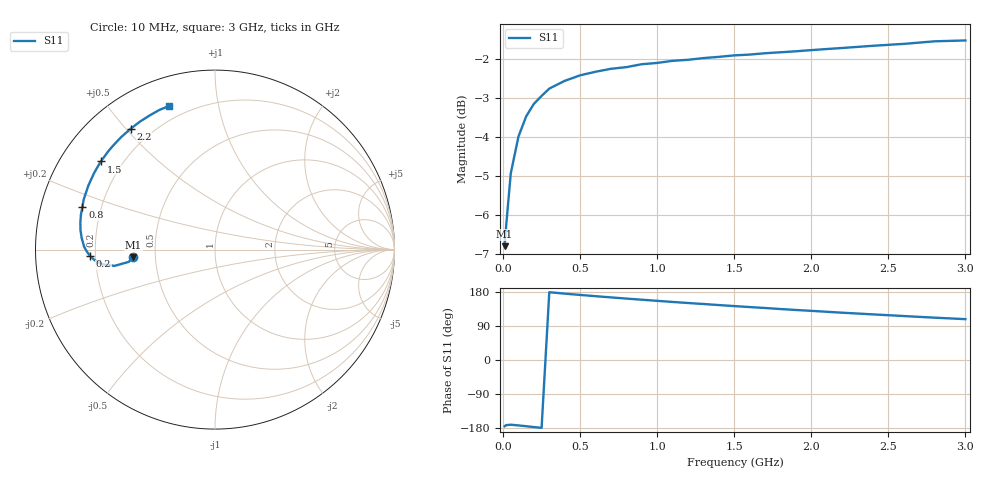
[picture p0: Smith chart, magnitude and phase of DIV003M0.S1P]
! SIEMENS Small Signal Semiconductors
! BAV99
! Silicon Switching Diode in SOT23
! IF = 3 mA
! S-Parameters:  May  1995
# GHz  S  MA  R  50
!  f  S11
! GHz  MAG  ANG
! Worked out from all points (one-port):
!   30 points, 10 MHz to 3 GHz, reference 50 ohm
!   lowest |S11| = -6.8 dB at 10 MHz (marker M1), VSWR 2.69, Z = 18.6 - j1.96 ohm
!   |S11| at or under -10 dB: nowhere
!   S11 on the Smith chart (normalised r, x): 10 MHz: 0.37, -0.04; 200 MHz: 0.18, -0.03; 800 MHz: 0.13, +0.15; 1.5 GHz: 0.12, +0.34; 2.2 GHz: 0.12, +0.52; 3 GHz: 0.13, +0.72
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0.01  0.4574 -174.8
0.02  0.4855 -171.9
0.05  0.5673 -170.8
0.1  0.6323 -172.6
0.15  0.6712 -174.8
0.2  0.6964 -177.0
0.25  0.7129 -179.0
0.3  0.7285 178.9
0.4  0.7453 175.1
0.5  0.7576 171.7
0.6  0.7657 168.4
0.7  0.7723 165.2
0.8  0.7762 162.1
0.9  0.7829 159.1
1.1  0.7908 153.2
1.2  0.7932 150.4
1.3  0.7972 147.8
1.5  0.8035 142.3
1.6  0.8055 139.7
1.7  0.8087 137.2
1.8  0.811 134.5
1.9  0.8133 132.0
2  0.8162 129.7
2.2  0.8213 124.8
2.4  0.8266 120.4
2.6  0.8313 116.0
2.8  0.8377 111.7
3  0.8398 107.8
